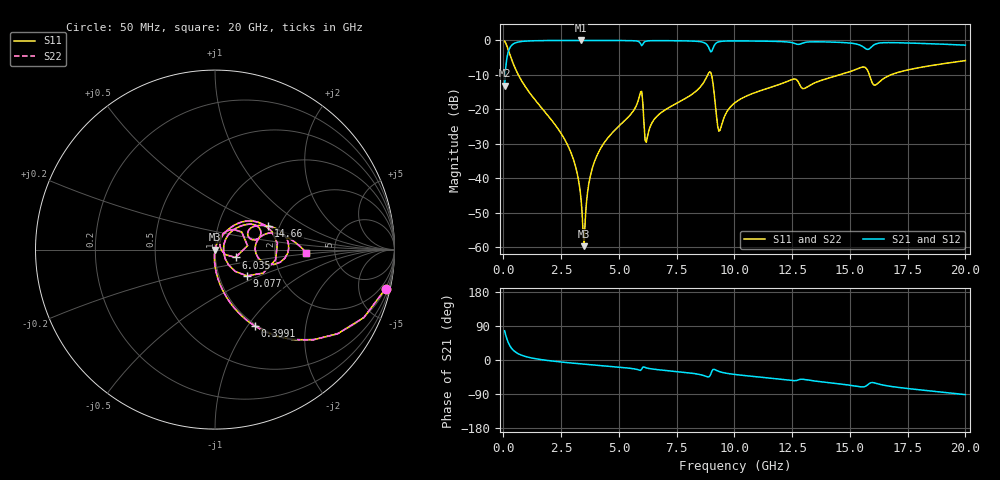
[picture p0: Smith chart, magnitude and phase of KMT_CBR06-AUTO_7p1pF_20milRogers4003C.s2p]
! Data measured by Modelithics Inc. support@modelithics.com 813-866-6335
! KEMET CBR06-AUTO 7.1pF, Pad Width= 0.851mm, Pad Length= 0.64mm, Pad Gap= 0.62mm, 20mil Rogers 4003C substrate Data, January 2022
# hz S ma R 50
! 2 Port Network Data from SP1.SP block
! freq  magS11  angS11  magS21  angS21  magS12  angS12  magS22  angS22
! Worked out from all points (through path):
!   401 points, 50 MHz to 20 GHz, reference 50 ohm
!   highest |S21| = -0.01 dB at 3.342 GHz (marker M1); lowest = -13.2 dB at 50 MHz (marker M2)
!   group delay of S21, straight-line fit = 14 ps
!   lowest |S11| = -59.8 dB at 3.491 GHz (marker M3), VSWR 1.00, Z = 50.1 + j0.0177 ohm
!   |S11| at or under -10 dB: 644.7 MHz to 8.844 GHz (8.2 GHz wide, 173 % of centre); 9.006 GHz to 14.56 GHz (5.555 GHz wide, 47.1 % of centre); 15.84 GHz to 16.77 GHz (929.7 MHz wide, 5.7 % of centre)
!   |S22| runs from -59.8 to -0.2 dB; largest |S21 - S12| = 0
!   S11 on the Smith chart (normalised r, x): 50 MHz: 0.98, -8.78; 399.1 MHz: 0.98, -1.09; 6.035 GHz: 1.25, -0.11; 9.077 GHz: 1.36, -0.42; 14.66 GHz: 1.74, +0.51; 20 GHz: 3.07, -0.15
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5e7  0.9755 -12.8  0.2196 77.1  0.2196 77.1  0.9755 -12.8
3.99125e8  0.4815 -62.4  0.8759 27.5  0.8759 27.5  0.4815 -62.4
2.74325e9  0.03188 -95.2  0.9985 -6.8  0.9985 -6.8  0.03188 -95.2
3.14225e9  0.01384 -95.3  0.9989 -9.1  0.9989 -9.1  0.01384 -95.3
3.34175e9  0.005643 -90.6  0.9989 -10.2  0.9989 -10.2  0.005643 -90.6
3.391625e9  0.003689 -85.6  0.9989 -10.4  0.9989 -10.4  0.003689 -85.6
3.491375e9  0.001027 9.9  0.9989 -11.0  0.9989 -11.0  0.001027 9.9
3.790625e9  0.01179 72.5  0.9988 -12.5  0.9988 -12.5  0.01179 72.5
4.13975e9  0.02456 73.1  0.9985 -14.4  0.9985 -14.4  0.02456 73.1
5.885375e9  0.1531 47.1  0.9466 -26.8  0.9466 -26.8  0.1531 47.1
6.035e9  0.1224 -20.9  0.8774 -18.6  0.8774 -18.6  0.1224 -20.9
6.2345e9  0.03994 47.2  0.9846 -21.6  0.9846 -21.6  0.03994 47.2
6.73325e9  0.08421 61.8  0.9927 -25.8  0.9927 -25.8  0.08421 61.8
8.72825e9  0.2653 36.8  0.9145 -42.2  0.9145 -42.2  0.2653 36.8
9.077375e9  0.2307 -39.4  0.7747 -24.9  0.7747 -24.9  0.2307 -39.4
9.376625e9  0.04961 14.2  0.9641 -31.1  0.9641 -31.1  0.04961 14.2
1.0025e10  0.1247 48.1  0.9839 -38.2  0.9839 -38.2  0.1247 48.1
1.336662e10  0.2325 31.1  0.9548 -54.6  0.9548 -54.6  0.2325 31.1
1.466338e10  0.3237 24.0  0.9336 -63.9  0.9336 -63.9  0.3237 24.0
1.58105e10  0.3395 -14.1  0.7441 -63.3  0.7441 -63.3  0.3395 -14.1
1.670825e10  0.3097 17.1  0.9296 -69.1  0.9296 -69.1  0.3097 17.1
2e10  0.5091 -2.0  0.8536 -91.3  0.8536 -91.3  0.5091 -2.0
